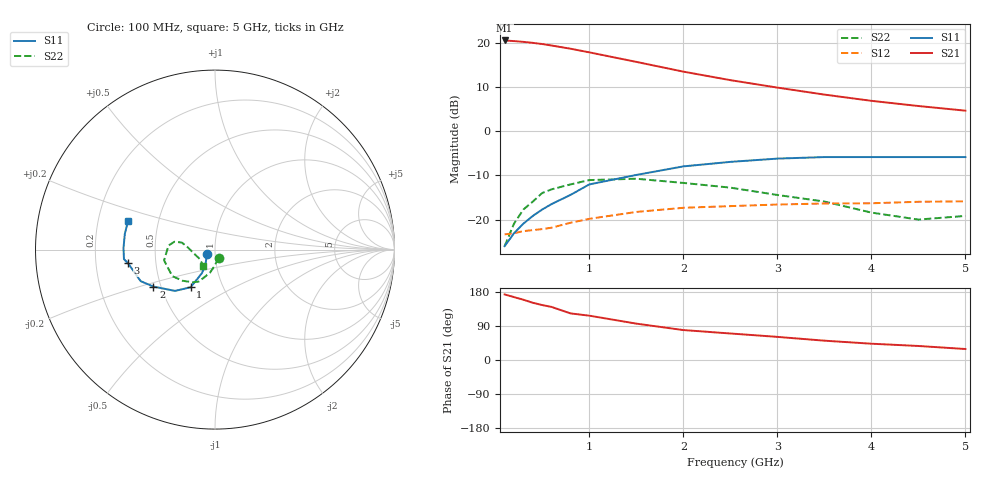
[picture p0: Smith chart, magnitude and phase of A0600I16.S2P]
!  MSA-0600 S AND NOISE PARAMETERS
!  Id=16mA  LAST UPDATED 07-22-92
# ghz s ma r 50
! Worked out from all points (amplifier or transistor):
!   16 points, 100 MHz to 5 GHz, reference 50 ohm
!   highest |S21| = 20.6 dB at 100 MHz (marker M1)
!   |S21| within 3 dB of that: start of sweep to 1.072 GHz
!   unconditionally stable (mu >= 1): start of sweep to 393.3 MHz; 2.778 GHz to end of sweep
!   at 300 MHz: K = 1.01, MAG = 20.7 dB, |S12| = -22.6 dB
!   at 1.5 GHz: K = 0.89, MSG = 17.0 dB, |S12| = -18.3 dB
!   at 5 GHz: K = 1.41, MAG = 6.4 dB, |S12| = -15.9 dB
!   lowest NFmin = 2.70 dB at 100 MHz
!   S11 on the Smith chart (normalised r, x): 100 MHz: 0.92, -0.05; 1 GHz: 0.70, -0.31; 2 GHz: 0.46, -0.22; 3 GHz: 0.34, -0.07; 5 GHz: 0.33, +0.14
0.1  0.05 -148.0  10.66 173.0  0.068 4.0  0.05 -67.0
0.2  0.07 -134.0  10.48 166.0  0.07 8.0  0.09 -91.0
0.3  0.09 -125.0  10.28 159.0  0.074 13.0  0.13 -102.0
0.4  0.11 -121.0  10.01 151.0  0.076 15.0  0.16 -110.0
0.5  0.13 -120.0  9.71 145.0  0.078 17.0  0.2 -117.0
0.6  0.15 -119.0  9.34 140.0  0.081 20.0  0.22 -124.0
0.8  0.19 -121.0  8.6 123.0  0.092 25.0  0.25 -136.0
1  0.25 -123.0  7.82 117.0  0.102 26.0  0.28 -148.0
1.5  0.32 -134.0  6.1 96.0  0.122 29.0  0.29 -168.0
2  0.4 -149.0  4.73 79.0  0.136 27.0  0.26 175.0
2.5  0.45 -157.0  3.79 70.0  0.142 30.0  0.23 169.0
3  0.49 -171.0  3.12 61.0  0.148 28.0  0.19 168.0
3.5  0.51 -174.0  2.6 51.0  0.152 25.0  0.16 173.0
4  0.51 179.0  2.21 43.0  0.153 26.0  0.12 -170.0
4.5  0.51 170.0  1.93 37.0  0.159 24.0  0.1 -149.0
5  0.51 162.0  1.71 29.0  0.161 24.0  0.11 -126.0
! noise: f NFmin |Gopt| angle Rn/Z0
0.1  2.7  0.11  5  0.39
0.5  2.8  0.1  25  0.39
1  3  0.09  53  0.38
2  3.3  0.1  127  0.35
